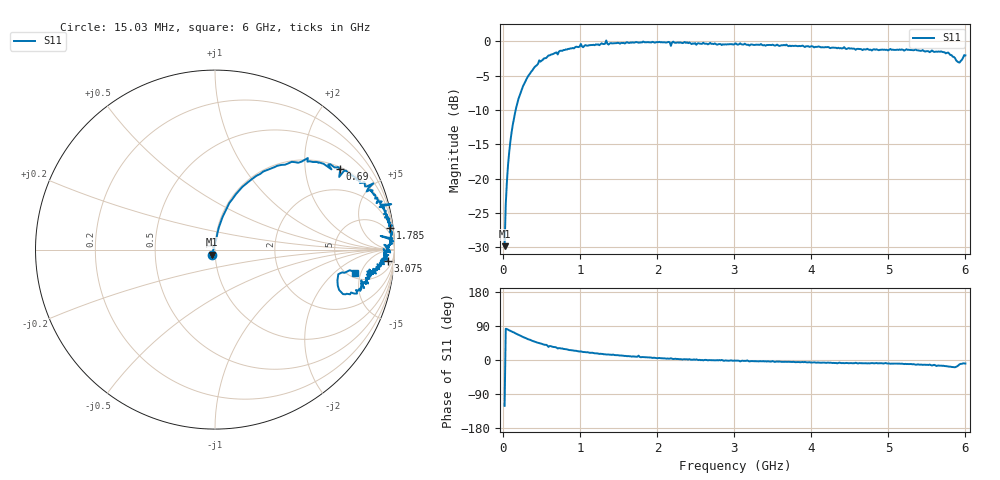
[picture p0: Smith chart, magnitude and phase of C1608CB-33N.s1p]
!	Network	Analyzer	HP8753E.07.74:	Oct	30	2002	Serial	No.	JP38451487
!	Hewlett-Packard
!	7	Sep	2009	9:43:19
!	Frequency	S11
#	HZ	S	RI	R	50
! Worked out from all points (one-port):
!   400 points, 15.03 MHz to 6 GHz, reference 50 ohm
!   lowest |S11| = -29.8 dB at 15.03 MHz (marker M1), VSWR 1.07, Z = 48.3 - j2.67 ohm
!   |S11| at or under -10 dB: start of sweep to 159 MHz
!   S11 on the Smith chart (normalised r, x): 15.03 MHz: 0.97, -0.05; 690 MHz: 1.07, +3.07; 1.785 GHz: 2, +16; 3.075 GHz: 12, -24; 6 GHz: 5.75, -3.94
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1.502992e7  -0.0166 -0.0276
3.002985e7  0.00854 0.0648
7.502962e7  0.0318 0.153
1.200294e8  0.068 0.235
1.95029e8  0.152 0.349
4.650277e8  0.517 0.51
6.900266e8  0.698 0.448
7.650262e8  0.735 0.43
1.320023e9  0.927 0.25
1.335023e9  0.982 0.253
1.365023e9  0.917 0.237
1.515022e9  0.941 0.198
1.755021e9  0.957 0.194
1.785021e9  0.974 0.123
2.145019e9  0.988 0.0611
2.175019e9  0.923 0.076
2.205019e9  0.993 0.0458
2.265019e9  0.981 0.0475
3.015015e9  0.966 -0.0301
3.075015e9  0.964 -0.0637
3.165014e9  0.941 -0.0162
3.765011e9  0.921 -0.0786
4.515007e9  0.879 -0.125
5.265004e9  0.853 -0.163
5.685002e9  0.816 -0.217
5.850001e9  0.728 -0.249
5.925e9  0.687 -0.137
6e9  0.779 -0.129
